| TEXAS INSTRUMENTS INCORPORATED
| Standard Linear and Logic Group
| IBIS Model of SN74CBTLV3857
| LOW-VOLTAGE 10-BIT FET BUS SWITCH WITH INTERNAL PULLDOWN RESISTORS
| This file contains package information for the following:
|  SOIC 24-pin (DW) package as [Component] CBTLV3857_DW
|  SSOP 24-pin (DBQ) package as [Component] CBTLV3857_DBQ
|  TVSOP 24-pin (DGV) package as [Component] CBTLV3857_DGV
|  TSSOP 24-pin (PW) package as [Component] CBTLV3857_PW
| This device can be powered at the following Vccs:
|  3.3 volt Vcc
| This file provides unique models under the [Model Selector] for each Vcc.
| For operation at a specific Vcc, select the appropriate model after each
| [Model Selector] keyword.
[IBIS Ver]   3.2
[Comment char]  |_char
[File Name]   sn74cbtlv3857.ibs
[File Rev]   1.1 | x_die
[Date]   July 14, 2003
[Source]   Data created from TI-SPICE simulations at TI-SLL.
[Notes]   The following is an IBIS list for the CBTLV3857.
   Please contact sllibis@ti.com with questions and
   comments concerning SLL IBIS models.
   - Power clamp data has been removed from VREF and AIO models.
   - Non-monotonic data due to FET characteristics.
   - Due to pullup resistor on BIO power clamp current never
   reaches zero.
   - Model selectors are include since A to B and B to A
   paths are different.
[Disclaimer] Property of Texas Instruments Incorporated.  Unauthorized
   reproduction and/or distribution is strictly prohibited.
   This product is protected under copyright law.
   Created  2003, (C) Copyright  2003, Texas Instruments
   Incorporated, All Rights Reserved
   UNLESS THERE IS A SIGNED, WRITTEN AGREEMENT TO THE
   CONTRARY, TEXAS INSTRUMENTS (TI) IS PROVIDING THE IBIS
   MODELS  AND WITHOUT ANY WARRANTY, EXPRESSED OR
   IMPLIED.  TI assumes no liability for:
   1) the accuracy of the IBIS models provided to your
   company;
   2) the proper functioning of these IBIS Models in your
   design or for any resulting applications; or
   3) infringement of patents, copyrights or intellectual
   property rights resulting from your use of these IBIS
   models.
   TI provides IBIS Models as a service to our customers.
   You and your company shall not distribute, sell or give
   these models to anyone else without prior written
   permission from TI.
   TI reserves the right to make changes to our products or
   to discontinue any semiconductor product or service
   without notice, and advises our customers to obtain the
   latest version of relevant information to verify, before
   placing orders, that the information being relied on is
   current.
   Please be aware that your receipt and use of the IBIS
   information provided shall serve as acceptance of these
   terms and conditions.  If you do not accept these terms,
   you should return or destroy the IBIS models and any
   other accompanying information immediately.
| Component CBTLV3857_DW 24-pin SOIC
[Component]   CBTLV3857_DW
[Manufacturer]   Texas Instruments, Inc.
[Package]
|   typ   min   max
R_pkg   3.700e-02   3.000e-02   4.700e-02
L_pkg   5.146e-09   3.993e-09   6.885e-09
C_pkg   7.580e-13   5.120e-13   1.067e-12
[Pin]   signal_name   model_name   R_pin   L_pin   C_pin
1   VREF   CBTLV3857_VREF   3.900e-02   6.885e-09   1.067e-12
2   A1   CBTLV3857_AIO   4.200e-02   5.950e-09   9.580e-13
3   A2   CBTLV3857_AIO   4.700e-02   5.317e-09   7.910e-13
4   A3   CBTLV3857_AIO   3.100e-02   4.651e-09   6.110e-13
5   A4   CBTLV3857_AIO   3.000e-02   3.993e-09   5.120e-13
6   A5   CBTLV3857_AIO   3.000e-02   4.083e-09   6.110e-13
7   A6   CBTLV3857_AIO   3.000e-02   4.083e-09   6.110e-13
8   A7   CBTLV3857_AIO   3.000e-02   3.993e-09   5.120e-13
9   A8   CBTLV3857_AIO   3.100e-02   4.652e-09   6.110e-13
10   A9   CBTLV3857_AIO   4.700e-02   5.317e-09   7.910e-13
11   A10   CBTLV3857_AIO   4.200e-02   5.950e-09   9.590e-13
12   GND   GND   3.900e-02   6.885e-09   1.067e-12
13   B10   CBTLV3857_BIO   3.900e-02   6.885e-09   1.067e-12
14   B9   CBTLV3857_BIO   4.200e-02   5.950e-09   9.590e-13
15   B8   CBTLV3857_BIO   4.700e-02   5.317e-09   7.910e-13
16   B7   CBTLV3857_BIO   3.100e-02   4.652e-09   6.110e-13
17   B6   CBTLV3857_BIO   3.000e-02   3.993e-09   5.120e-13
18   B5   CBTLV3857_BIO   3.000e-02   4.083e-09   6.100e-13
19   B4   CBTLV3857_BIO   3.000e-02   4.083e-09   6.100e-13
20   B3   CBTLV3857_BIO   3.000e-02   3.993e-09   5.120e-13
21   B2   CBTLV3857_BIO   3.100e-02   4.651e-09   6.110e-13
22   B1   CBTLV3857_BIO   4.700e-02   5.317e-09   7.910e-13
23   NOE   CBTLV3857_NOE   4.200e-02   5.950e-09   9.580e-13
24   VCC   POWER   3.900e-02   6.885e-09   1.067e-12
| Component CBTLV3857_DBQ 24-pin SSOP
[Component]   CBTLV3857_DBQ
[Manufacturer]   Texas Instruments, Inc.
[Package]
|   typ   min   max
R_pkg   4.400e-02   3.100e-02   6.600e-02
L_pkg   3.074e-09   2.348e-09   4.044e-09
C_pkg   3.220e-13   2.340e-13   4.460e-13
[Pin]   signal_name   model_name   R_pin   L_pin   C_pin
1   VREF   CBTLV3857_VREF   6.500e-02   4.044e-09   4.290e-13
2   A1   CBTLV3857_AIO   6.600e-02   3.824e-09   4.460e-13
3   A2   CBTLV3857_AIO   3.100e-02   3.011e-09   3.210e-13
4   A3   CBTLV3857_AIO   3.200e-02   2.699e-09   2.590e-13
5   A4   CBTLV3857_AIO   3.500e-02   2.519e-09   2.450e-13
6   A5   CBTLV3857_AIO   3.500e-02   2.348e-09   2.340e-13
7   A6   CBTLV3857_AIO   3.500e-02   2.348e-09   2.340e-13
8   A7   CBTLV3857_AIO   3.500e-02   2.518e-09   2.450e-13
9   A8   CBTLV3857_AIO   3.200e-02   2.699e-09   2.590e-13
10   A9   CBTLV3857_AIO   3.100e-02   3.011e-09   3.210e-13
11   A10   CBTLV3857_AIO   6.600e-02   3.824e-09   4.460e-13
12   GND   GND   6.500e-02   4.044e-09   4.290e-13
13   B10   CBTLV3857_BIO   6.500e-02   4.044e-09   4.290e-13
14   B9   CBTLV3857_BIO   6.600e-02   3.824e-09   4.460e-13
15   B8   CBTLV3857_BIO   3.100e-02   3.011e-09   3.210e-13
16   B7   CBTLV3857_BIO   3.200e-02   2.699e-09   2.590e-13
17   B6   CBTLV3857_BIO   3.500e-02   2.518e-09   2.450e-13
18   B5   CBTLV3857_BIO   3.500e-02   2.348e-09   2.340e-13
19   B4   CBTLV3857_BIO   3.500e-02   2.348e-09   2.340e-13
20   B3   CBTLV3857_BIO   3.500e-02   2.518e-09   2.450e-13
21   B2   CBTLV3857_BIO   3.200e-02   2.699e-09   2.590e-13
22   B1   CBTLV3857_BIO   3.100e-02   3.011e-09   3.210e-13
23   NOE   CBTLV3857_NOE   6.600e-02   3.824e-09   4.460e-13
24   VCC   POWER   6.500e-02   4.044e-09   4.290e-13
| Component CBTLV3857_DGV 24-pin TVSOP
[Component]   CBTLV3857_DGV
[Manufacturer]   Texas Instruments, Inc.
[Package]
|   typ   min   max
R_pkg   4.300e-02   3.900e-02   4.700e-02
L_pkg   2.601e-09   2.312e-09   3.626e-09
C_pkg   3.580e-13   2.770e-13   5.950e-13
[Pin]   signal_name   model_name   R_pin   L_pin   C_pin
1   VREF   CBTLV3857_VREF   4.300e-02   3.625e-09   5.950e-13
2   A1   CBTLV3857_AIO   4.000e-02   2.656e-09   4.020e-13
3   A2   CBTLV3857_AIO   3.900e-02   2.338e-09   3.080e-13
4   A3   CBTLV3857_AIO   4.600e-02   2.354e-09   2.770e-13
5   A4   CBTLV3857_AIO   4.500e-02   2.312e-09   2.850e-13
6   A5   CBTLV3857_AIO   4.700e-02   2.318e-09   2.820e-13
7   A6   CBTLV3857_AIO   4.700e-02   2.318e-09   2.820e-13
8   A7   CBTLV3857_AIO   4.500e-02   2.312e-09   2.850e-13
9   A8   CBTLV3857_AIO   4.600e-02   2.353e-09   2.780e-13
10   A9   CBTLV3857_AIO   3.900e-02   2.338e-09   3.080e-13
11   A10   CBTLV3857_AIO   4.100e-02   2.660e-09   4.020e-13
12   GND   GND   4.300e-02   3.625e-09   5.950e-13
13   B10   CBTLV3857_BIO   4.400e-02   3.626e-09   5.940e-13
14   B9   CBTLV3857_BIO   4.000e-02   2.658e-09   4.020e-13
15   B8   CBTLV3857_BIO   3.900e-02   2.343e-09   3.110e-13
16   B7   CBTLV3857_BIO   4.600e-02   2.353e-09   2.780e-13
17   B6   CBTLV3857_BIO   4.500e-02   2.312e-09   2.850e-13
18   B5   CBTLV3857_BIO   4.700e-02   2.319e-09   2.820e-13
19   B4   CBTLV3857_BIO   4.700e-02   2.319e-09   2.820e-13
20   B3   CBTLV3857_BIO   4.500e-02   2.312e-09   2.850e-13
21   B2   CBTLV3857_BIO   4.600e-02   2.353e-09   2.780e-13
22   B1   CBTLV3857_BIO   3.900e-02   2.337e-09   3.080e-13
23   NOE   CBTLV3857_NOE   4.000e-02   2.658e-09   4.020e-13
24   VCC   POWER   4.400e-02   3.626e-09   5.950e-13
| Component CBTLV3857_PW 24-pin TSSOP
[Component]   CBTLV3857_PW
[Manufacturer]   Texas Instruments, Inc.
[Package]
|   typ   min   max
R_pkg   3.900e-02   3.000e-02   4.600e-02
L_pkg   2.685e-09   2.367e-09   3.177e-09
C_pkg   3.200e-13   2.520e-13   4.340e-13
[Pin]   signal_name   model_name   R_pin   L_pin   C_pin
1   VREF   CBTLV3857_VREF   3.700e-02   3.153e-09   4.340e-13
2   A1   CBTLV3857_AIO   3.400e-02   2.629e-09   3.410e-13
3   A2   CBTLV3857_AIO   3.200e-02   2.860e-09   3.470e-13
4   A3   CBTLV3857_AIO   4.200e-02   2.741e-09   2.900e-13
5   A4   CBTLV3857_AIO   4.600e-02   2.600e-09   2.620e-13
6   A5   CBTLV3857_AIO   4.300e-02   2.414e-09   2.660e-13
7   A6   CBTLV3857_AIO   4.200e-02   2.367e-09   2.620e-13
8   A7   CBTLV3857_AIO   4.400e-02   2.461e-09   2.520e-13
9   A8   CBTLV3857_AIO   4.200e-02   2.543e-09   2.740e-13
10   A9   CBTLV3857_AIO   3.000e-02   2.616e-09   3.320e-13
11   A10   CBTLV3857_AIO   3.700e-02   2.670e-09   3.460e-13
12   GND   GND   3.900e-02   3.177e-09   4.330e-13
13   B10   CBTLV3857_BIO   3.700e-02   3.111e-09   4.310e-13
14   B9   CBTLV3857_BIO   3.700e-02   2.656e-09   3.450e-13
15   B8   CBTLV3857_BIO   3.100e-02   2.739e-09   3.400e-13
16   B7   CBTLV3857_BIO   4.200e-02   2.649e-09   2.820e-13
17   B6   CBTLV3857_BIO   4.600e-02   2.532e-09   2.570e-13
18   B5   CBTLV3857_BIO   4.400e-02   2.425e-09   2.660e-13
19   B4   CBTLV3857_BIO   4.400e-02   2.425e-09   2.660e-13
20   B3   CBTLV3857_BIO   4.600e-02   2.532e-09   2.570e-13
21   B2   CBTLV3857_BIO   4.200e-02   2.648e-09   2.820e-13
22   B1   CBTLV3857_BIO   3.100e-02   2.738e-09   3.390e-13
23   NOE   CBTLV3857_NOE   3.600e-02   2.653e-09   3.440e-13
24   VCC   POWER   3.700e-02   3.110e-09   4.310e-13
[Series Switch Groups]
| Function Group States
On  1 /   | A1-A10->B1-B10 NOE LOW
Off 1 /   | NOE HIGH
[Series Pin Mapping]   pin_2   model_name   function_table_group
2   22   CBTLV3857_AIO_S   1
| 2   22   CBTLV3857_BIO_S   1
3   21   CBTLV3857_AIO_S   1
| 3   21   CBTLV3857_BIO_S   1
4   20   CBTLV3857_AIO_S   1
| 4   20   CBTLV3857_BIO_S   1
5   19   CBTLV3857_AIO_S   1
| 5   19   CBTLV3857_BIO_S   1
6   18   CBTLV3857_AIO_S   1
| 6   18   CBTLV3857_BIO_S   1
7   17   CBTLV3857_AIO_S   1
| 7   17   CBTLV3857_BIO_S   1
8   16   CBTLV3857_AIO_S   1
| 8   16   CBTLV3857_BIO_S   1
9   15   CBTLV3857_AIO_S   1
| 9   15   CBTLV3857_BIO_S   1
10   14   CBTLV3857_AIO_S   1
| 10   14   CBTLV3857_BIO_S   1
11   13   CBTLV3857_AIO_S   1
| 11   13   CBTLV3857_BIO_S   1
| Model CBTLV3857_IO_S
[Model Selector]   CBTLV3857_IO_S
CBTLV3857_AIO_S   Series-Switch Model for A->B Path
CBTLV3857_BIO_S   Series-Switch Model for B->A Path
[Model]   CBTLV3857_BIO_S
Model_type  Series_switch
| variable   typ   min   max
C_comp   0   0   0
[Temperature Range]   40   100   -40
| Ambient temperature   25   85   -40
[Voltage range]   3.3   3   3.6
[On]
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[Off]
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[Model]   CBTLV3857_AIO_S
Model_type  Series_switch
| variable   typ   min   max
C_comp   0   0   0
[Temperature Range]   40   100   -40
| Ambient temperature   25   85   -40
[Voltage range]   3.3   3   3.6
[On]
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[Off]
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| Models and submodels in the file (6): CBTLV3857_VREF (Input), CBTLV3857_NOE (Input), CBTLV3857_BIO_S (Series_switch), CBTLV3857_BIO (Terminator), CBTLV3857_AIO_S (Series_switch), CBTLV3857_AIO (Terminator)
